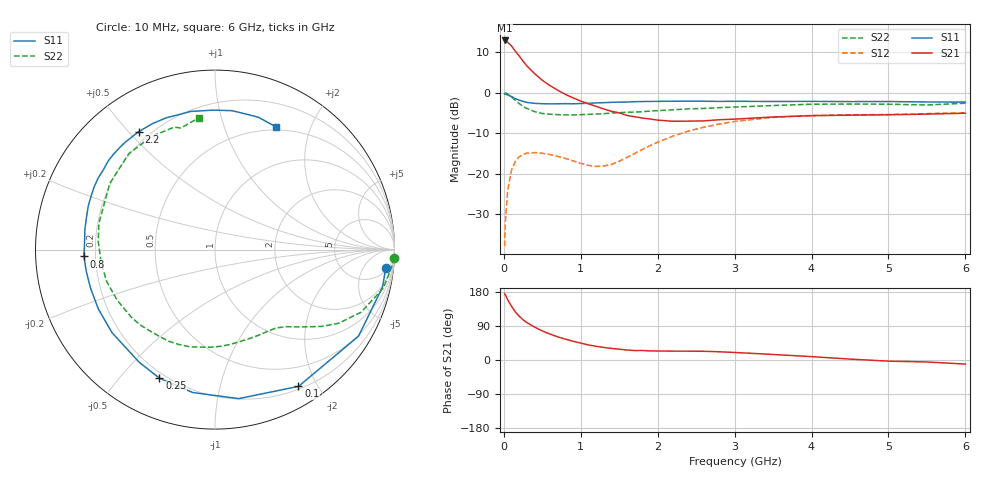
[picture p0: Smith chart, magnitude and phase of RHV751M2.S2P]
! SIEMENS Small Signal Semiconductors
! BFR106
! Si NPN RF Bipolar Junction Transistor in SOT23
! VCE = 0.75 V  IC = 1.2 mA
! Common Emitter S-Parameters:  August  1996
# GHz  S  MA  R  50
!  f  S11  S21  S12  S22
! GHz  MAG  ANG  MAG  ANG  MAG  ANG  MAG  ANG
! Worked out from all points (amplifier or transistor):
!   36 points, 10 MHz to 6 GHz, reference 50 ohm
!   highest |S21| = 12.9 dB at 10 MHz (marker M1)
!   |S21| within 3 dB of that: start of sweep to 164.1 MHz
!   unconditionally stable (mu >= 1): 816.5 MHz to end of sweep
!   at 250 MHz: K = 0.30, MSG = 11.5 dB, |S12| = -15.2 dB
!   at 1.4 GHz: K = 1.54, MAG = 2.2 dB, |S12| = -17.7 dB
!   at 6 GHz: K = 1.02, MAG = -1.0 dB, |S12| = -5.0 dB
!   S11 on the Smith chart (normalised r, x): 10 MHz: 6, -16; 100 MHz: 0.23, -1.76; 250 MHz: 0.18, -0.64; 800 MHz: 0.16, -0.03; 2.2 GHz: 0.16, +0.53; 6 GHz: 0.46, +1.52
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0.01  0.9566 -6.3  4.392 175.2  0.0128 87.6  0.9981 -2.6
0.02  0.9565 -12.6  4.358 171.8  0.0255 85.4  0.9904 -5.3
0.05  0.9339 -31.1  4.169 159.0  0.0621 71.6  0.9629 -12.8
0.1  0.8928 -58.6  3.753 142.1  0.1111 57.0  0.8857 -23.2
0.15  0.8407 -81.0  3.23 126.7  0.1427 44.4  0.8017 -30.8
0.2  0.8058 -98.9  2.822 115.7  0.1618 35.9  0.7332 -35.7
0.25  0.7803 -113.4  2.44 106.0  0.173 28.7  0.6734 -39.7
0.3  0.7567 -123.9  2.133 98.8  0.1795 24.0  0.6377 -42.5
0.4  0.7372 -141.1  1.713 86.7  0.1822 16.4  0.5825 -47.5
0.5  0.7294 -153.0  1.419 76.7  0.1788 11.7  0.5529 -52.3
0.6  0.726 -162.6  1.219 68.4  0.1723 8.6  0.5412 -57.4
0.8  0.7312 -177.0  0.95 55.0  0.1544 7.1  0.5314 -68.6
1.1  0.7379 166.1  0.727 39.7  0.1267 17.1  0.5398 -86.6
1.3  0.7515 156.8  0.628 33.0  0.1247 31.2  0.5498 -98.8
1.6  0.7647 144.3  0.523 26.3  0.1587 49.6  0.5724 -117.0
2.2  0.7827 122.9  0.443 23.4  0.2913 52.4  0.6136 -152.5
2.8  0.7787 105.0  0.463 21.7  0.4095 39.8  0.6522 176.1
3.5  0.7772 90.6  0.501 14.6  0.4951 24.2  0.6927 147.8
4.5  0.7748 76.9  0.527 2.4  0.533 6.3  0.7223 118.9
5  0.776 71.8  0.533 -3.0  0.5366 -0.2  0.7191 108.4
5.5  0.7663 66.8  0.543 -5.2  0.551 -3.3  0.7035 105.7
6  0.764 63.4  0.557 -10.8  0.5649 -9.9  0.7396 97.0
